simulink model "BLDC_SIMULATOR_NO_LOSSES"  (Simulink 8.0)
settings: Solver=ode45  StartTime=0.0  StopTime=10  FixedStep=0.0000001  RelTol=1e-6  AbsTol=1e-6
undefined symbols (not defined in the file): CA, Fr, H_Freq, J, Kd, Ki, Kp, Kv, L, LoopFreq, P, PAM, PWM, R, Vs
libraries: simulink x4, powerlib_extras x1

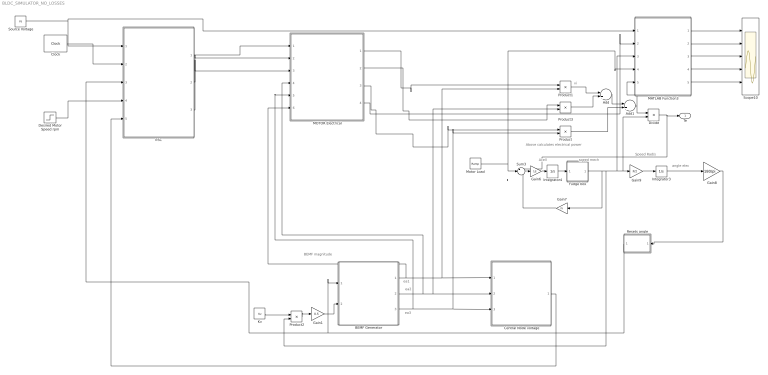
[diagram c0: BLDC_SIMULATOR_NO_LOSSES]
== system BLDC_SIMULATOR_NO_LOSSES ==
  note: Above calculates electrical power
  note: ea1
  note: ea2
  note: ea3
  note: vi
  note: Acell
  note: Speed Rad/s
  note: angle elec
  note: BEMF magnitude
  note: Tl
  note: speed mech
  Add : Sum
  Add1 : Sum
  BEMF Generator : MATLAB Function  TreatAsAtomicUnit=on
  Central Node voltage : MATLAB Function  TreatAsAtomicUnit=on
  Clock : Clock
  Desired Motor Speed rpm : Step  Time=0.5  Before=4e64  After=35000  SampleTime=0
  Divide : Product  Inputs=*/
  ESC : Subsystem
  Fudge box : MATLAB Function  TreatAsAtomicUnit=on
  Gain1 : Gain  Gain=0.5
  Gain6 : Gain  Gain=1/J
  Gain7 : Gain  Gain=Fr
  Gain8 : Gain  Gain=180/pi
  Gain9 : Gain  Gain=P/2
  Integrator3 : Integrator
  Integrator4 : Integrator  InitialCondition=0.00001
  Kv : Constant  Value=Kv
  MATLAB Function3 : MATLAB Function  TreatAsAtomicUnit=on
  MOTOR Electrical : Subsystem
  Motor Load : simulink/Sources/Ramp  slope=0  start=0  X0=0
  Product{,1..3} (4 alike) : Product
  Resets angle : MATLAB Function  TreatAsAtomicUnit=on
  Scope10 : Scope  NumInputPorts=5
  Source Voltage : Constant  Value=Vs
  Sum3 : Sum  Inputs=+--
  Te : Outport
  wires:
  Product1/1 -> Add/1
  Product3/1 -> Add/2
  Add/1 -> Add1/1
  Product/1 -> Add1/2
  Kv/1 -> Product2/1
  Product2/1 -> Gain1/1
  BEMF Generator/1(y1) -> MOTOR Electrical/6(ea), Central Node voltage/1(u4), Product1/2
  BEMF Generator/2(y2) -> MOTOR Electrical/4(eb), Product3/2, Central Node voltage/2(u5)
  BEMF Generator/3(y3) -> MOTOR Electrical/5(ec), Product/2, Central Node voltage/3(u6)
  Integrator4/1 -> Fudge box/1(u1)
  Gain6/1 -> Integrator4/1
  Sum3/1 -> Gain6/1
  Gain7/1 -> Sum3/3
  Integrator3/1 -> Gain8/1
  Divide/1 -> Sum3/1, Te/1
  Resets angle/1(yd) -> ESC/3(angle elec), BEMF Generator/1(u1)
  Add1/1 -> Divide/1, MATLAB Function3/5(u5)
  Gain8/1 -> Resets angle/1(ud)
  Gain9/1 -> Integrator3/1
  MATLAB Function3/1(y1) -> Scope10/1
  MATLAB Function3/2(y2) -> Scope10/2
  MATLAB Function3/3(y3) -> Scope10/3
  MATLAB Function3/4(y4) -> Scope10/4
  MATLAB Function3/5(y5) -> Scope10/5
  MOTOR Electrical/1(Ia) -> Product1/1
  MOTOR Electrical/3(Ic) -> Product/1
  MOTOR Electrical/2(Ib) -> Product3/1
  Source Voltage/1 -> MATLAB Function3/1(u1), ESC/1(V batt)
  Clock/1 -> ESC/2(Clock)
  MOTOR Electrical/4(I-Avg) -> MATLAB Function3/2(u2)
  Gain1/1 -> BEMF Generator/2(u2)
  Desired Motor Speed rpm/1 -> ESC/4(Ref Speed)
  Fudge box/1(y1) -> MATLAB Function3/3(u3), Divide/2, Gain9/1, Product2/2, Gain7/1
  Central Node voltage/1(y) -> ESC/5(Central node voltage)
  ESC/1(Va) -> MOTOR Electrical/1(In1)
  ESC/2(Vb) -> MOTOR Electrical/2(In2)
  ESC/3(Vc) -> MOTOR Electrical/3(In3)
  Motor Load/1 -> Sum3/2, MATLAB Function3/4(u4)

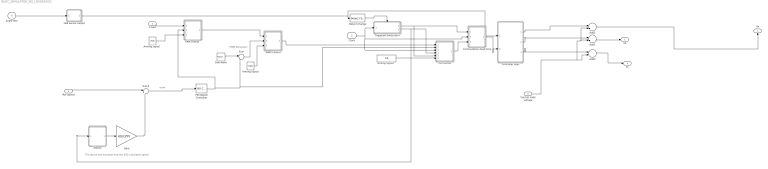
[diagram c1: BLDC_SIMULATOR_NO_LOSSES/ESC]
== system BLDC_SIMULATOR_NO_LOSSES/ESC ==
  note: The above two simulate how the ESC calculates speed
  note: PWM Generator
  note: error
  V batt : Inport
  Clock : Inport  Port=2
  angle elec : Inport  Port=3
  Ref Speed : Inport  Port=4
  Central node voltage : Inport  Port=5
  Add1 : Sum  Inputs=+-
  Add2 : Sum  Inputs=+-
  Add3 : Sum  Inputs=+-
  Arming Signal : Constant  Value=PWM
  "Arming signal  " : Constant  Value=PAM
  "Arming signal   " : Constant  Value=CA
  CA Control : MATLAB Function  TreatAsAtomicUnit=on
  Commutation dead time : MATLAB Function  TreatAsAtomicUnit=on
  Controller logic : MATLAB Function  TreatAsAtomicUnit=on
  Detect Change : simulink/Logic and Bit Operations/Detect Change  vinit=64  InputProcessing=Inherited  OutDataTypeStr=boolean
  Gain : Gain  Gain=60/(3*P)
  Hall sensor output : MATLAB Function  TreatAsAtomicUnit=on
  "PAM control  " : MATLAB Function  TreatAsAtomicUnit=on
  PID Speed Controller : simulink/Continuous/PID Controller  Controller=PID  TimeDomain=Discrete-time  SampleTime=1/LoopFreq  IntegratorMethod=Trapezoidal  FilterMethod=Forward Euler  Form=Parallel  P=Kp  I=Ki  D=Kd  N=100  InitialConditionSource=internal  InitialConditionForIntegrator=0.4  InitialConditionForFilter=0  ExternalReset=none  LimitOutput=on  UpperSaturationLimit=1  LowerSaturationLimit=0  LinearizeAsGain=off  AntiWindupMode=none  Kb=1  TrackingMode=off  Kt=1  PParamMin=[]  PParamMax=[]  IParamMin=[]  IParamMax=[]  DParamMin=[]  DParamMax=[]  NParamMin=[]  NParamMax=[]  KbParamMin=[]  KbParamMax=[]  KtParamMin=[]  KtParamMax=[]  POutMin=[]  POutMax=[]  IOutMin=[]  IOutMax=[]  DOutMin=[]  DOutMax=[]  NOutMin=[]  NOutMax=[]  KbOutMin=[]  KbOutMax=[]  KtOutMin=[]  KtOutMax=[]  IntegratorOutMin=[]  IntegratorOutMax=[]  FilterOutMin=[]  FilterOutMax=[]  SumOutMin=[]  SumOutMax=[]  SumI1OutMin=[]  SumI1OutMax=[]  SumI2OutMin=[]  SumI2OutMax=[]  SumI3OutMin=[]  SumI3OutMax=[]  SumDOutMin=[]  SumDOutMax=[]  SaturationOutMin=[]  SaturationOutMax=[]  IntegratorContinuousStateAttributes=''  IntegratorStateMustResolveToSignalObject=off  IntegratorRTWStateStorageClass=Auto  FilterContinuousStateAttributes=''  FilterStateMustResolveToSignalObject=off  FilterRTWStateStorageClass=Auto
  PWM Control : MATLAB Function  TreatAsAtomicUnit=on
  Saw Wave : simulink/Sources/Repeating Sequence  rep_seq_t=[0 1/H_Freq]  rep_seq_y=[0 1]
  Starter : MATLAB Function  TreatAsAtomicUnit=on
  Sum : Sum  Inputs=|-+
  Sum4 : Sum  Inputs=|+-
  Triggered Subsystem : Subsystem  TreatAsAtomicUnit=on
  Va : Outport
  Vb : Outport  Port=2
  Vc : Outport  Port=3
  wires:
  angle elec/1 -> Hall sensor output/1(u1)
  Clock/1 -> Commutation dead time/2(u2), CA Control/3(u3), Triggered Subsystem/1(In1)
  Sum4/1 -> PID Speed Controller/1
  Ref Speed/1 -> Sum4/1
  PWM Control/1(y) -> CA Control/1(u1)
  Saw Wave/1 -> Sum/1
  Arming Signal/1 -> PWM Control/3(u3)
  Hall sensor output/1(y1) -> Controller logic/1(u1), Detect Change/1
  Detect Change/1 -> Triggered Subsystem/Trigger
  V batt/1 -> "PAM control  "/1(u1)
  "PAM control  "/1(y) -> PWM Control/1(u1)
  "Arming signal  "/1 -> "PAM control  "/3(u3)
  "Arming signal   "/1 -> CA Control/6(u6)
  Triggered Subsystem/2(Out2) -> CA Control/4(u4), Starter/1(u1)
  Triggered Subsystem/1(Out1) -> Commutation dead time/1(u1), CA Control/5(u5)
  Starter/1(y) -> Gain/1
  Gain/1 -> Sum4/2
  PID Speed Controller/1 -> CA Control/2(u2), Sum/2, "PAM control  "/2(u2)
  Central node voltage/1 -> Add3/2, Add2/2, Add1/2
  Controller logic/1(y1) -> Add2/1
  Controller logic/2(y2) -> Add1/1
  Controller logic/3(y3) -> Add3/1
  CA Control/1(y) -> Commutation dead time/3(u3)
  Commutation dead time/1(y) -> Controller logic/2(u2)
  Sum/1 -> PWM Control/2(u2)
  Add2/1 -> Va/1
  Add1/1 -> Vb/1
  Add3/1 -> Vc/1

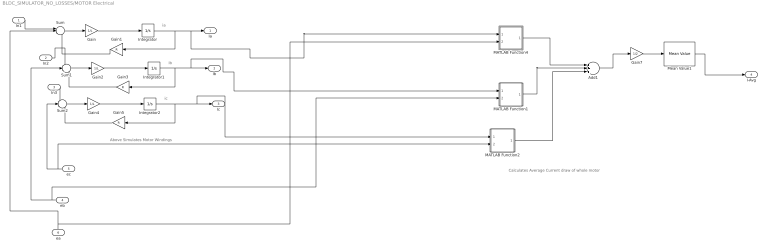
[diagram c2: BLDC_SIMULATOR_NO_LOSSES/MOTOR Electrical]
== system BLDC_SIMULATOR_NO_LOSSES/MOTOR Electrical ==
  note: Calculates Average Current draw of whole motor
  note: Above Simulates Motor Windings
  note: i'
  note: ia
  note: i'
  note: ib
  note: i'
  note: ic
  In1 : Inport
  In2 : Inport  Port=2
  In3 : Inport  Port=3
  eb : Inport  Port=4
  ec : Inport  Port=5
  ea : Inport  Port=6
  Add1 : Sum  Inputs=+++
  Gain : Gain  Gain=1/L
  Gain1 : Gain  Gain=R
  Gain2 : Gain  Gain=1/L
  Gain3 : Gain  Gain=R
  Gain4 : Gain  Gain=1/L
  Gain5 : Gain  Gain=R
  Gain7 : Gain  Gain=1/2
  Integrator : Integrator
  Integrator1 : Integrator
  Integrator2 : Integrator
  MATLAB Function1 : MATLAB Function  TreatAsAtomicUnit=on
  MATLAB Function2 : MATLAB Function  TreatAsAtomicUnit=on
  MATLAB Function4 : MATLAB Function  TreatAsAtomicUnit=on
  Mean Value1 : powerlib_extras/Measurements/Mean Value  Period=1/1000
  Sum : Sum  Inputs=+--
  Sum1 : Sum  Inputs=+--
  Sum2 : Sum  Inputs=+--
  Ia : Outport
  Ib : Outport  Port=2
  Ic : Outport  Port=3
  I-Avg : Outport  Port=4
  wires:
  In2/1 -> Sum1/1
  ea/1 -> MATLAB Function4/2(u2), Sum/2
  In1/1 -> Sum/1
  eb/1 -> MATLAB Function1/2(u2), Sum1/2
  ec/1 -> MATLAB Function2/2(u2), Sum2/2
  In3/1 -> Sum2/1
  Sum1/1 -> Gain2/1
  Gain3/1 -> Sum1/3
  Gain/1 -> Integrator/1
  Gain5/1 -> Sum2/3
  Integrator2/1 -> MATLAB Function2/1(u1), Ic/1, Gain5/1
  Sum/1 -> Gain/1
  Integrator/1 -> MATLAB Function4/1(u1), Ia/1, Gain1/1
  Gain4/1 -> Integrator2/1
  Gain1/1 -> Sum/3
  Gain2/1 -> Integrator1/1
  Integrator1/1 -> MATLAB Function1/1(u1), Ib/1, Gain3/1
  Sum2/1 -> Gain4/1
  Add1/1 -> Gain7/1
  Mean Value1/1 -> I-Avg/1
  MATLAB Function2/1(y1) -> Add1/3
  MATLAB Function1/1(y1) -> Add1/2
  MATLAB Function4/1(y1) -> Add1/1
  Gain7/1 -> Mean Value1/1

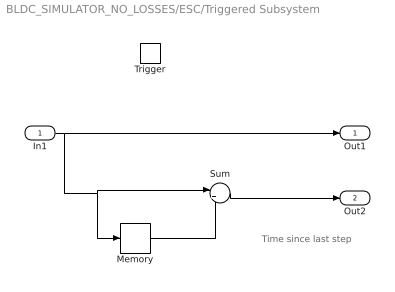
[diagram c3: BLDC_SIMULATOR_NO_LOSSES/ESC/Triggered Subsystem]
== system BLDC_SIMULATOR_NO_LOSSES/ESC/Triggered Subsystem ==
  note: Time since last step
  In1 : Inport
  Trigger : TriggerPort
  Memory : Memory  X0=-1  InheritSampleTime=on
  Sum : Sum  Inputs=|+-
  Out1 : Outport
  Out2 : Outport  Port=2
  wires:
  In1/1 -> Out1/1, Memory/1, Sum/1
  Sum/1 -> Out2/1
  Memory/1 -> Sum/2

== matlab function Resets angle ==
function yd = fcn(ud)

 if  ud<360
        yd=ud;
    else  
        yd=mod(ud,360)
     end

end
 % Makes sure angle starts over when it reaches 360 [ makes life easier
 % later on]

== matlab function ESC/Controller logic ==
function [y1,y2,y3]= ESC(u1,u2)
    %%u1 is pposition ,
    %u2 is source voltage. 
  
   
 E=(u2/2); % sets voltage of batters to each phase assuming ballanced its just batt Volt divided by two
 El=-E;
 Eo=0;
    

               
                                                                   if u1==1  %%List of if statments to generate input voltages [ logic]

                                                                                            y1=E;
                                                                                            y2=El;
                                                                                            y3=0;

                                                                                        else if u1==2
                                                                                            y1=E;
                                                                                            y2=0;
                                                                                            y3=El;

                                                                                        else if u1==3
                                                                                            y1=0;
                                                                                            y2=E;
                                                                                            y3=El;


                                                                                        else if u1==4
                                                                                            y1=El;
                                                                                            y2=E;
                                                                                            y3=0;


                                                                                        else if u1==5
                                                                                            y1=El;
                                                                                            y2=0;
                                                                                            y3=E;


                                                                                        else if u1==6
                                                                                            y1=0;
                                                                                            y2=El;
                                                                                            y3=E;


                                                                                        else  
                                                                                            y1=0;
                                                                                            y2=0;
                                                                                            y3=0;

                                                                                            end
                                                                                            end
                                                                                            end
                                                                                            end
                                                                                            end
                                                                   end
                                                         
                 
end

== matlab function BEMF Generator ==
function [y1,y2,y3] = BEMF(u1,u2) %%Declaring inputs and outputs
% Caluculate BEMF for each phase
    if 0<=u1 && u1<60   %%List of if statments to generate BEMF of trapeziodal shape 
        y1=u2; %%Top of trapeziode 
	  y3=(((6*u2)/180)*(60-(u1)))-u2; 
	  y2=-u2;

	else if 60<=u1 && u1<120
y1=u2;
y3=-u2;
y2=((((6*u2)/180))*((u1)-(120)))+u2;

    else if 120<=u1 && u1<180
y1=(((6*u2)/180)*(180-(u1)))-u2; 
y3=-u2;
y2=u2;


	else if 180<=u1 && u1<240
y1=-u2;
y3=((((6*u2)/180))*((u1)-(240)))+u2;
y2=u2;

 
    else if 240<=u1 && u1<300
y1=-u2;  
y3=u2;
y2=(((6*u2)/180)*(300-(u1)))-u2; 
 


    else if 300<=u1 && u1<361
y1=((((6*u2)/180))*((u1)-(360)))+u2;
y3=u2;
y2=-u2;

					 
  else
y1=1000000000;
y2=1000000000;
y3=1000000000; 

        end
        end
        end
        end
        end
        
        
    end

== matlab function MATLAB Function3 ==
function [y1,y2,y3,y4,y5]  = fcn(u1,u2,u3,u4,u5)
%#codegen
Vs=u1;
Ibus=u2;
Wm=u3;
Tl=u4;
Pelec=u5;


% working out electrical power in
Pin = Vs*Ibus;
y1=Pin;

% working out useful mechanical power out
Pmech=Wm*Tl;

y2=Pmech;

% Total effcieicny
Teff= ((Pmech/Pin)*100);
y3=Teff;


% Input power to electomagentic torqe efficiency 

y4= (Pelec/Pin)*100;

% Mech effcieincy 

y5=((Pmech/Pelec)*100);

% controller Losses








end

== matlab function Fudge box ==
function y1 = ESC(u1)

% Stops simulator from quiting if zero motor speed is reached, fudge factor
% employed set a minimum speed of a miniscule amount, shouldnt cause
% problems with results.

      
   

  

            if u1>0  
                y1=u1;
               
          

            else  
               y1=0.000000000000000001;

                end
               
                
                
end

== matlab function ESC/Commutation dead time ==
function y =  ESD(u1,u2,u3)
   
    %u1= time of last step
    %u2=actual time
 
    
    % Impliments dead time between commutation step to prevent shoot thru
       
   
 
 

 if (u2-u1)>2e-6
      y=u3;
              
 else 
     y=0;
     
 end
                
                
end

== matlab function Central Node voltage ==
function y  = BEMF(u4,u5,u6) %%Declaring inputs and outputs

%Calculates central node voltage for star type stator
%u4=ea
%u5=eb
%u6=ec
%u7= step
   
   y=(-u4-u5-u6);
  
   
    end

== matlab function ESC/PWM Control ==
function y = ESC(u1,u2,u3)
    %u1= Source voltage
    %u2= PWM waveform
    %u3 = PWM simulator arming signal
   
    
    
         
            if u2<0 && u3>0.5
                y=0;
                
                              
            
                
                        else  
                y=u1;
               

                end
                
                
end

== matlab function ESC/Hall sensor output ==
function y1  = ESC(u1)
    
% This Code Simulates the Hall sensors, asigning a value of one to 6
% depending upon rotor position
                
                                if (0)<=u1 && u1<(60)  
                                    y1=1;
                                   
                                  

                                else if (60)<=u1 && u1<(120)
                                    y1=2;
                                 
                                   

                                else if (120)<=u1 && u1<(180)
                                    y1=3;
                                   


                                else if (180)<=u1 && u1<(240)
                                    y1=4;
                             


                                else if (240)<=u1 && u1<(300)
                                    y1=5;
                                 

                                else if (300)<=u1 && u1<=(360)
                                    y1=6;
                                 


                                else  
                                    y1=0; % used for error checking
                                   
                                    end
                                    end
                                    end
                                    end
                                    end
                                    
                                    
                                end
 
 
                
end

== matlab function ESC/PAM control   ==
function y = ESC(u1,u2,u3)
    %u1= Source voltage
    %u2= PAM duty cycle
    %u3 = PAM simulator arming signal
   % Impliments PAM by reducing Buss bar voltage
       
         
            if u3>0.5
                y=u1*u2;
                            
            
                
                        else  
                y=u1;
               

                end
                
                
end

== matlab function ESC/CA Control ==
function y = ESC(u1,u2,u3,u4,u5,u6)
    %u1 is source voltage
    %u2 is comutation angle feed back [o= full power, 60 = no power]      
    %u3 is the main time
    %u4 commutation time period
    %u5= time of last step
    %u6= PAM arming signal
    
    
       
   
 
 

 if u6>0.5 %checks if CA is being simulated, if not just pass thru value
      StepTime= u4;
    
                       if u2 ==1 
                                         Tdelay=  -0.05;
                                       %this just makes sure it powers the phase for long enough during
                                     %speeding the rotor up, but still has inherant saftey protection if
                                       %locked rotor happens

                       else 
                                     Tdelay= (StepTime)*(1-u2);

                       end
                       
                    
                                        
                                       


                                                                                              if u3>=(u5+Tdelay)  && u3<=(u5+0.1);  %decides if angle is in conduction period
                                                                                                  y=u1;

                                                                                              else
                                                                                                  y=0;

                                                                                              end
                                                                                              
                                        
              
 else 
     y=u1;
                
                
end

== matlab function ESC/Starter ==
function y = ESC(u1)
    % simulates how ESC caculates speed,  1/ last step time
         
            if u1==0  % to stop an infinate error
                y=10;
                            
            
                
                        else  
                y=(1/u1);
               

                end
                
                
end

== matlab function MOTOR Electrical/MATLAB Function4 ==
function y1 = ESC(u1,u2)
   

      % these boxes check that the current is of the same polarity of the
      %  current will be negative under breaking etc.
   

  

            if u1>0 && u2>0  
                y1=u1;
               
          

            else  if  u1<0 && u2<0
y1=-u1;
else

        y1=-abs(u1);
                end
end
               
                
                
end

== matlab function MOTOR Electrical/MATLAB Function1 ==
function y1 = ESC(u1,u2)
    %%u1 is pposition , u2 is source voltage.

      
   

  

            if u1>0 && u2>0  %%List of if statments to generate input voltages [ logic]
                y1=u1;
               
          

            else if  u1<0 && u2<0
                y1=-u1;
else

                y1=-abs(u1);
                end
end
               
                
                
end

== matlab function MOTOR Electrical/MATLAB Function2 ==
function y1 = ESC(u1,u2)
    %%u1 is pposition , u2 is source voltage.

      
   

  

            if u1>0 && u2>0  %%List of if statments to generate input voltages [ logic]
                y1=u1;
               
          

            else  if  u1<0 && u2<0
y1=-u1;
else

       y1=-abs(u1);
                end
end
               
                
                
end
